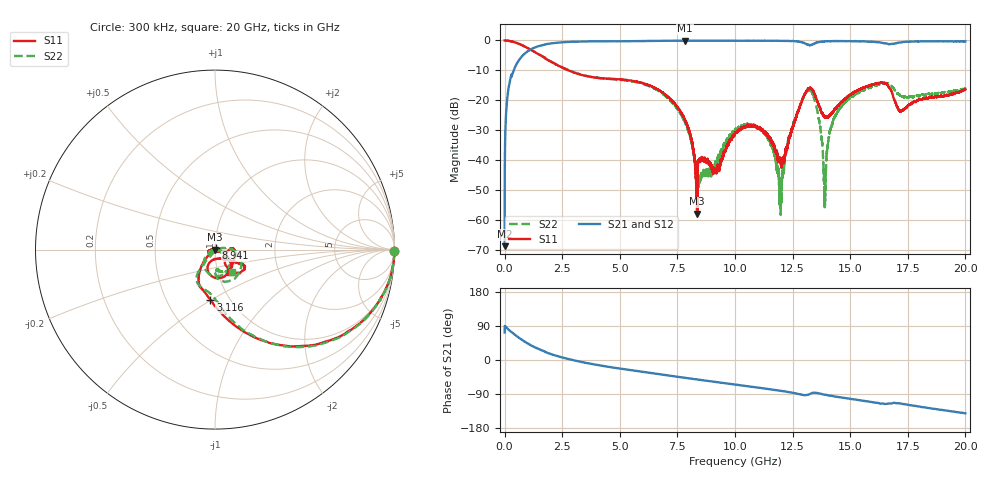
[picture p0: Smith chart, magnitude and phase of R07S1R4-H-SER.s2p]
!{R07S1R4}
!Johanson Technology Inc.
!www.johansontechnology.com
!Test Board Conditions:
!Substrate Type  RO4350B
!Substrate Thickness  10 mil
!Substrate Dk  3.66
!TL Type: GCPW
!TL Trace Width  21 mil
!TL Gap  20 mil
!Electrode orientation  Horizontal
!DUT TOPOLOGY	SERIES
!Mounting Pad LxW  16x21 mil
! Created Sat Feb  6 11:18:34 2021
# hz S ma R 50
! 2 Port Network Data from SP1.SP block
! freq  magS11  angS11  magS21  angS21  magS12  angS12  magS22  angS22
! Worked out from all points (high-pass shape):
!   20001 points, 300 kHz to 20 GHz, reference 50 ohm
!   highest |S21| = -0.05 dB at 7.829 GHz (marker M1); lowest = -68.8 dB at 300 kHz (marker M2)
!   |S21| within 3 dB of the highest: 1.125 GHz to end of sweep
!   lowest |S11| = -57.9 dB at 8.363 GHz (marker M3), VSWR 1.00, Z = 50.1 - j0.114 ohm
!   |S11| at or under -10 dB: 2.764136 GHz to 2.767229 GHz (3.094 MHz wide, 0.112 % of centre); 2.76736 GHz to 2.770176 GHz (2.816 MHz wide, 0.102 % of centre); 2.77 GHz to end of sweep
!   |S22| runs from -58.3 to 0.0 dB; largest |S21 - S12| = 0.012
!   S11 on the Smith chart (normalised r, x): 300 kHz: open; 3.116 GHz: 0.82, -0.50; 8.941 GHz: 1.01, +0.02; 20 GHz: 1.14, -0.29
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300000  0.9995 -0.5  0.0003635 72.3  0.0002812 83.2  1 -0.6
1.313e8  0.9914 -7.6  0.122 82.5  0.122 82.6  0.9923 -7.8
4.843e8  0.9209 -24.4  0.38 65.1  0.3797 65.0  0.9231 -24.7
1.8243e9  0.485 -70.6  0.8686 19.6  0.8687 19.7  0.4876 -69.4
3.1163e9  0.2817 -95.1  0.9556 -2.4  0.9541 -2.4  0.2848 -88.6
3.3343e9  0.266 -98.3  0.9604 -5.2  0.9598 -5.2  0.2688 -91.1
6.6673e9  0.1503 -124.7  0.9844 -36.9  0.9845 -37.0  0.1443 -127.2
7.8293e9  0.04669 -139.6  0.9942 -47.0  0.9925 -47.0  0.04271 -126.6
8.3633e9  0.001267 -63.7  0.9922 -51.5  0.9939 -51.5  0.006692 -36.8
8.9413e9  0.008831 64.0  0.9912 -56.2  0.9921 -56.2  0.005824 -40.5
1.00003e10  0.02796 -171.9  0.9929 -64.8  0.9922 -64.9  0.03069 -139.5
1.12953e10  0.02979 -156.9  0.9877 -75.3  0.9878 -75.4  0.02745 -162.1
1.19943e10  0.009358 -101.7  0.9866 -81.4  0.986 -81.5  0.002472 -99.7
1.24993e10  0.03469 -22.2  0.9805 -86.6  0.9788 -86.5  0.03555 -13.1
1.33343e10  0.1548 -92.5  0.8485 -87.3  0.8476 -87.4  0.1368 -105.5
1.36443e10  0.08108 -113.6  0.9421 -88.3  0.9422 -88.3  0.04722 -150.1
1.39033e10  0.05285 -90.8  0.9651 -91.5  0.9655 -91.5  0.00176 91.6
1.41583e10  0.05847 -60.5  0.9745 -94.5  0.9749 -94.5  0.03336 14.0
1.45793e10  0.09002 -39.9  0.9757 -98.6  0.9756 -98.6  0.0756 5.4
1.66673e10  0.1684 -49.6  0.8661 -114.8  0.8685 -115.2  0.1893 -70.5
1.72003e10  0.06602 -24.0  0.9255 -115.0  0.9299 -115.1  0.1153 -87.6
2e10  0.1508 -56.1  0.9641 -140.7  0.9595 -140.7  0.1576 -53.1
